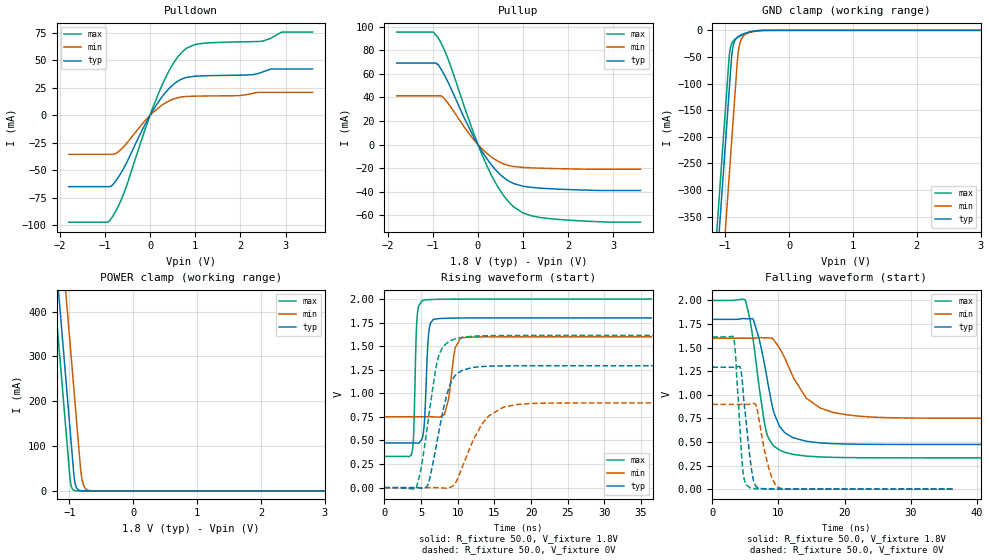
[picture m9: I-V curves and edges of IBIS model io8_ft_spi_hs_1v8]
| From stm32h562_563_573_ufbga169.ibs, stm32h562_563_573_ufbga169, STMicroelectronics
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[Model]   io8_ft_spi_hs_1v8
Model_type I/O
Polarity   Non-Inverting
Enable   Active-Low
| CAP_THRESHOLD on pad IOFT is "UDTCAPC" :
| Rising=20.0% of vddiom   Falling=80.0% of vddiom
| C_comp min and max val. don't necessarily correlate with the min and max pvt
| but are the smallest and greatest pad capacitance found.
| var   typ   min   max
C_comp   4.56197pF  4.45395pF  4.75009pF
|C_comp_pullup   2.85120pF  2.67105pF  2.77155pF
|C_comp_pulldown   1.71077pF  1.78290pF  1.97854pF
Vinl = 480.0mV
Vinh = 1.4V
Vmeas = 900.0mV   | Reference voltage for timing measurements
Cref  = 50.0pF   | Timing specification test load capacitance value
Rref  = 100.0MOhm   | Timing specification test load resistance value
Vref  = 900.0mV   | Timing specification test load voltage
[Model Spec]
| TIME_THRESHOLD on pin ZIV11 is "CMOS" :
| Rising=40.0% of vdd   Falling=60.0% of vdd
Vinl 703.80000mV 631.80000mV 784.80000mV
Vinh 1.06220V 937.20000mV 1.16620V
| variable   typ   min   max
[Temperature Range] 25.0 125.0 -40.0
| variable   typ   min   max
[Voltage Range] 1.8V 1.6V 2.0V
| variable   typ   min   max
[POWER Clamp Reference] 1.8V 1.6V 2.0V
| variable   typ   min   max
[GND Clamp Reference] 0V 0V 0V
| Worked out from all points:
|   slope of the pulldown table from 0 to 0.27 V, typ, clamps not added: 15.8 ohm
|   slope of the pullup table from 0 to 0.27 V, typ, clamps not added: 17.2 ohm
|   GND clamp passes 1 mA (typ) near -0.52 V on its own axis
|   POWER clamp passes 1 mA (typ) near -0.84 V on its own axis
|   rising waveform, R_fixture 50.0, V_fixture 1.8V: 20-80 % time 445ps typ, 841ps min, 330ps max; typ from 0.474 V to 1.8 V
|   falling waveform, R_fixture 50.0, V_fixture 1.8V: 20-80 % time 2.46ns typ, 4.42ns min, 2ns max; typ from 1.8 V to 0.474 V
|   rising waveform, R_fixture 50.0, V_fixture 0V: 20-80 % time 2.09ns typ, 3.35ns min, 1.83ns max; typ from 0 V to 1.29 V
|   falling waveform, R_fixture 50.0, V_fixture 0V: 20-80 % time 1.18ns typ, 1.63ns min, 840ps max; typ from 1.29 V to 0 V
[POWER Clamp]
-1.8V     1.518A     1.709A     1.407A
-1.23V    548.8mA    740.2mA    437.5mA
-1.16V    429.8mA    621.2mA    318.5mA
-1.05V    242.8mA    434.2mA    131.5mA
-980mV    123.8mA    315.2mA    17.95mA
-930mV    38.81mA    230.2mA    1.49mA
-910mV    17.82mA    196.2mA    550.8uA
-890mV    8.18mA     162.2mA    203.5uA
-810mV    363.5uA    33.6mA     3.797uA
-770mV    76.62uA    10.47mA    518.8nA
-710mV    7.417uA    1.822mA    26.38nA
3.6V      0A         0A         0A
[GND Clamp]
-1.8V     -1.581A    -1.742A    -1.516A
-1.24V    -628.8mA   -789.9mA   -564.1mA
-1.05V    -305.8mA   -466.9mA   -241.1mA
-940mV    -118.8mA   -279.9mA   -54.1mA
-930mV    -101.8mA   -262.9mA   -41.86mA
-900mV    -51.51mA   -211.9mA   -25.34mA
-880mV    -32.22mA   -177.9mA   -21mA
-810mV    -13.02mA   -59.5mA    -13.82mA
-770mV    -9.8mA     -24.99mA   -11mA
-680mV    -5.275mA   -7.288mA   -5.917mA
-400mV    -107uA     -349.1uA   -42.51uA
3.6V      5.392nA    968.2nA    261.3pA
| variable   typ   min   max
[Pullup Reference] 1.8V 1.6V 2.0V
| variable   typ   min   max
[Pulldown Reference] 0V 0V 0V
[Pullup]
-1.8V     69.08mA    41.34mA    95.3mA
-990mV    69.08mA    41.34mA    95.3mA
-880mV    67.7mA     41.34mA    90.21mA
-790mV    62.19mA    40.81mA    84.08mA
-660mV    52.71mA    34.79mA    72.3mA
-120mV    8.364mA    5.386mA    12.19mA
190mV     -11.56mA   -7.18mA    -17.34mA
500mV     -25.61mA   -15.24mA   -39.45mA
810mV     -33.32mA   -18.7mA    -53.33mA
1.18V     -36.29mA   -19.75mA   -60.37mA
1.56V     -37.38mA   -20.24mA   -62.7mA
3.6V      -38.97mA   -20.89mA   -65.81mA
[Pulldown]
-1.8V     -65.02mA   -35.56mA   -97.42mA
-940mV    -65.02mA   -35.56mA   -97.42mA
-850mV    -64.17mA   -35.56mA   -93.5mA
-570mV    -47.32mA   -28.01mA   -70.04mA
-120mV    -9.088mA   -5.279mA   -14.07mA
250mV     16.04mA    8.832mA    26.05mA
550mV     29.17mA    15.25mA    49.41mA
780mV     34.17mA    17.07mA    60.14mA
1.18V     35.97mA    17.56mA    65.65mA
2.49V     39.44mA    20.93mA    67.53mA
2.92V     42.19mA    20.93mA    75.82mA
3.6V      42.19mA    20.93mA    75.82mA
[Ramp]
dV/dt_r 775.81164mV/2.08546ns 538.94795mV/3.30173ns 968.32208mV/1.83296ns
dV/dt_f 795.78721mV/2.40354ns 508.98204mV/4.21025ns 1.00099V/1.99569ns
R_load = 50.0
| Removed startup time: 0s 0s 0s  .
| Removed end time: 36.4ns.
[Rising Waveform]
R_fixture   = 50.0
V_fixture   = 1.8V
V_fixture_min = 1.6V
V_fixture_max = 2.0V
0s        473.7mV    751.7mV    331.7mV
3.75ns    473.7mV    751.7mV    370.2mV
4ns       473.6mV    751.7mV    604mV
4.45ns    471.5mV    751.7mV    1.803V
5.15ns    519.4mV    751.7mV    1.982V
6ns       1.605V     751.8mV    1.994V
6.7ns     1.785V     751.3mV    1.996V
8.2ns     1.796V     777.6mV    1.998V
10.4ns    1.799V     1.587V     2V
36.4ns    1.8V       1.6V       2V
| Removed startup time: 0s 0s 0s  .
| Removed end time: 99.4ns.
[Falling Waveform]
R_fixture   = 50.0
V_fixture   = 1.8V
V_fixture_min = 1.6V
V_fixture_max = 2.0V
0s        1.8V       1.6V       2V
4.95ns    1.807V     1.6V       2.007V
6.2ns     1.794V     1.6V       1.568V
8.3ns     1.165V     1.604V     577.1mV
9.25ns    828.6mV    1.586V     461.3mV
10.15ns   667.6mV    1.498V     415.3mV
12.2ns    546.1mV    1.193V     368.9mV
16.25ns   490.8mV    862.5mV    341.8mV
22.35ns   476.2mV    773mV      333.4mV
99.4ns    473.7mV    751.7mV    331.7mV
| Removed startup time: 0s 0s 0s  .
| Removed end time: 99.3ns.
[Rising Waveform]
R_fixture   = 50.0
V_fixture   = 0V
V_fixture_min = 0V
V_fixture_max = 0V
0s        134.8nV    547.1nV    93.87nV
4.3ns     232uV      1.933uV    -9.838mV
5ns       -5.887mV   762.5nV    207.3mV
5.9ns     25.76mV    2.574uV    676mV
7.5ns     624.2mV    -529.4uV   1.417V
8.8ns     1.058V     -2.401mV   1.547V
10.1ns    1.219V     116.5mV    1.586V
14.2ns    1.288V     759.1mV    1.612V
18.3ns    1.292V     883.7mV    1.614V
99.3ns    1.293V     898.2mV    1.614V
| Removed startup time: 0s 0s 0s  .
| Removed end time: 36.4ns.
[Falling Waveform]
R_fixture   = 50.0
V_fixture   = 0V
V_fixture_min = 0V
V_fixture_max = 0V
0s        1.293V     898.3mV    1.614V
3.2ns     1.293V     898.3mV    1.608V
3.5ns     1.293V     898.3mV    1.431V
4.2ns     1.291V     898.3mV    609.9mV
4.6ns     1.084V     898.3mV    206.3mV
5.7ns     329.7mV    900.5mV    15.09mV
6.6ns     29.56mV    891.3mV    4.779mV
8.2ns     3.631mV    316.2mV    1.742mV
9.65ns    1.856mV    28.3mV     952.7uV
36.4ns    217.3nV    4.053uV    206.5nV
